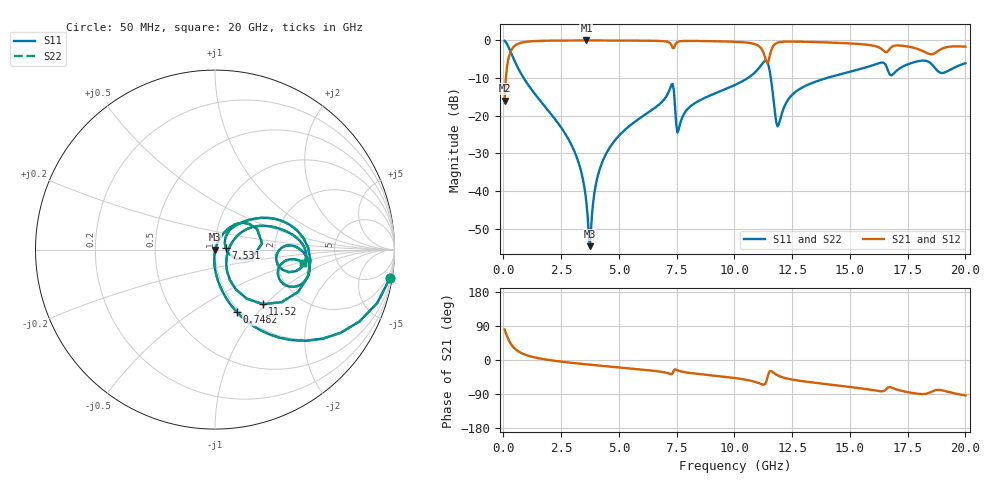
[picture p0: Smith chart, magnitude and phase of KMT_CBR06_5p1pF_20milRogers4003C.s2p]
! Data measured by Modelithics Inc. support@modelithics.com 813-866-6335
! KEMET CBR0603 5.1pF, Pad Width= 0.851mm, Pad Length= 0.64mm, Pad Gap= 0.62mm, 20mil Rogers 4003C substrate Data, January 2022
# hz S ma R 50
! 2 Port Network Data from SP1.SP block
! freq  magS11  angS11  magS21  angS21  magS12  angS12  magS22  angS22
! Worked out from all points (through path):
!   401 points, 50 MHz to 20 GHz, reference 50 ohm
!   highest |S21| = -0.02 dB at 3.591 GHz (marker M1); lowest = -15.9 dB at 50 MHz (marker M2)
!   group delay of S21, straight-line fit = 15.3 ps
!   lowest |S11| = -54.6 dB at 3.741 GHz (marker M3), VSWR 1.00, Z = 50.2 - j0.0152 ohm
!   |S11| at or under -10 dB: 878.9 MHz to 10.57 GHz (9.695 GHz wide, 169 % of centre); 11.58 GHz to 13.99 GHz (2.412 GHz wide, 18.9 % of centre)
!   |S22| runs from -54.6 to -0.1 dB; largest |S21 - S12| = 0
!   S11 on the Smith chart (normalised r, x): 50 MHz: 1, -12; 748.2 MHz: 0.97, -0.78; 7.531 GHz: 1.12, +0.03; 11.52 GHz: 1.33, -0.96; 20 GHz: 2.86, -0.55
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5e7  0.9872 -9.3  0.1595 80.6  0.1595 80.6  0.9872 -9.3
2.99375e8  0.7163 -45.2  0.697 44.8  0.697 44.8  0.7163 -45.2
7.4825e8  0.3694 -70.7  0.9283 19.2  0.9283 19.2  0.3694 -70.7
2.74325e9  0.05334 -94.3  0.9969 -6.0  0.9969 -6.0  0.05334 -94.3
3.391625e9  0.01681 -94.3  0.998 -10.3  0.998 -10.3  0.01681 -94.3
3.591125e9  0.007085 -86.7  0.998 -11.5  0.998 -11.5  0.007085 -86.7
3.74075e9  0.001866 -4.6  0.998 -12.4  0.998 -12.4  0.001866 -4.6
4.04e9  0.01398 67.9  0.9978 -14.2  0.9978 -14.2  0.01398 67.9
4.488875e9  0.03324 69.7  0.9972 -16.8  0.9972 -16.8  0.03324 69.7
6.73325e9  0.1406 57.3  0.984 -30.3  0.984 -30.3  0.1406 57.3
7.281875e9  0.2611 25.7  0.8545 -37.5  0.8545 -37.5  0.2611 25.7
7.53125e9  0.06004 11.2  0.9518 -26.9  0.9518 -26.9  0.06004 11.2
1.0025e10  0.2569 40.5  0.9581 -47.7  0.9581 -47.7  0.2569 40.5
1.107238e10  0.4335 19.2  0.8333 -61.5  0.8333 -61.5  0.4335 19.2
1.132175e10  0.5356 -6.6  0.6015 -63.7  0.6015 -63.7  0.5356 -6.6
1.152125e10  0.4035 -48.8  0.6089 -30.2  0.6089 -30.2  0.4035 -48.8
1.187038e10  0.07232 -15.8  0.9334 -40.4  0.9334 -40.4  0.07232 -15.8
1.246888e10  0.1854 33.3  0.9646 -51.2  0.9646 -51.2  0.1854 33.3
1.336662e10  0.2727 28.7  0.952 -59.2  0.952 -59.2  0.2727 28.7
1.630925e10  0.5046 -0.9  0.7919 -82.5  0.7919 -82.5  0.5046 -0.9
1.670825e10  0.3595 -13.5  0.7613 -71.5  0.7613 -71.5  0.3595 -13.5
2e10  0.4977 -8.3  0.8259 -93.5  0.8259 -93.5  0.4977 -8.3
